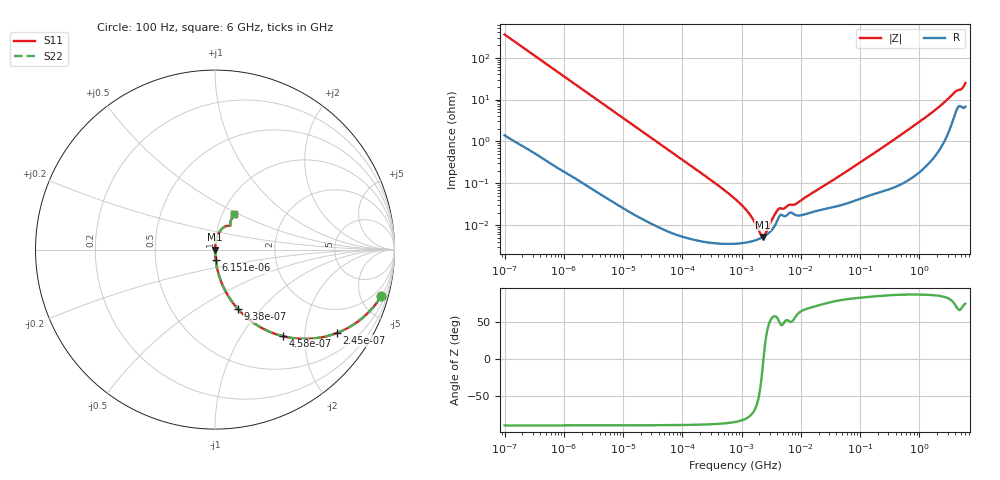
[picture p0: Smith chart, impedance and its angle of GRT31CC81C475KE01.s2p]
!Murata Part Number: GRT31CC81C475KE01
!These Parameters are Measured in Series Mode Connection
!Data Generated on Jun 19, 2026
!  o--ll--o
!Port1  Port2
!  o------o
!Operation Temp=25[degC], DC Bias Voltage=0[V]
!Freq. Start=100[Hz] Stop=6[GHz] 401[Steps]
# Hz S RI R 50
!Freq.(Hz) S11(Real) S11(Imag) S21(Real) S21(Imag) S12(Real) S12(Imag) S22(Real) S22(Imag)
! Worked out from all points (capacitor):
!   401 points, 100 Hz to 6 GHz, reference 50 ohm
!   read as one part in series: C = 4.45 uF near 109 Hz
!   lowest |Z| = 5.26 mohm at 2.269 MHz (marker M1)
!   series resonance near 2.342 MHz, so ESL is about 1 nH
!   S11 on the Smith chart (normalised r, x): 100 Hz: 1.03, -7.15; 245 Hz: 1.01, -2.93; 458 Hz: 1.01, -1.57; 938 Hz: 1.00, -0.77; 6.151 kHz: 1.00, -0.12; 6 GHz: 1.13, +0.48
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100  0.9265 -0.259  0.0735 0.259  0.0735 0.259  0.9265 -0.259
164  0.8259 -0.3771  0.1741 0.3771  0.1741 0.3771  0.8259 -0.3771
245  0.6807 -0.464  0.3193 0.464  0.3193 0.464  0.6807 -0.464
458  0.3806 -0.4831  0.6194 0.4831  0.6194 0.4831  0.3806 -0.4831
938  0.1294 -0.333  0.8706 0.333  0.8706 0.333  0.1294 -0.333
2008  0.0322 -0.1736  0.9678 0.1736  0.9678 0.1736  0.0322 -0.1736
6151  0.00384 -0.0586  0.9962 0.0586  0.9962 0.0586  0.00384 -0.0586
40335  0.00017 -0.00904  0.9998 0.00904  0.9998 0.00904  0.00017 -0.00904
316350  3.88e-05 -0.00114  1 0.00114  1 0.00114  3.88e-05 -0.00114
774597  3.62e-05 -0.000424  1 0.000424  1 0.000424  3.62e-05 -0.000424
1212075  3.86e-05 -0.000223  1 0.000223  1 0.000223  3.86e-05 -0.000223
1734173  4.37e-05 -9.65e-05  1 9.65e-05  1 9.65e-05  4.37e-05 -9.65e-05
2268635  5.16e-05 -1.01e-05  0.9999 1.01e-05  0.9999 1.01e-05  5.16e-05 -1.01e-05
2967816  6.75e-05 7.79e-05  0.9999 -7.79e-05  0.9999 -7.79e-05  6.75e-05 7.79e-05
4246196  0.000154 0.000192  0.9998 -0.000192  0.9998 -0.000192  0.000154 0.000192
8311524  0.000173 0.000274  0.9998 -0.000274  0.9998 -0.000274  0.000173 0.000274
1.555665e7  0.000205 0.000548  0.9998 -0.000548  0.9998 -0.000548  0.000205 0.000548
3.124326e8  0.000805 0.00919  0.9992 -0.00919  0.9992 -0.00919  0.000805 0.00919
1.873145e9  0.00772 0.0561  0.9923 -0.0561  0.9923 -0.0561  0.00772 0.0561
3.8344e9  0.0524 0.1263  0.9476 -0.1263  0.9476 -0.1263  0.0524 0.1263
5.016141e9  0.0848 0.1364  0.9152 -0.1364  0.9152 -0.1364  0.0848 0.1364
6e9  0.1075 0.1993  0.8925 -0.1993  0.8925 -0.1993  0.1075 0.1993
